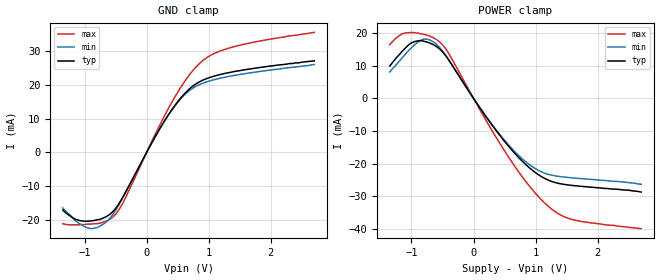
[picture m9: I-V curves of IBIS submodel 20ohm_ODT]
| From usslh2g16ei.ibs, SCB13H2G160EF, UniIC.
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| SUBMODEL 20ohm_ODT
[Submodel]   20ohm_ODT
Submodel_type  Dynamic_clamp
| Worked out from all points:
|   GND clamp passes 1 mA (typ) near -0.03 V on its own axis
[GND Clamp]
|Voltage   I(typ)   I(min)   I(max)
-1.35V    -17.1mA    -16.5mA    -21.15mA
-1.15V    -19.8mA    -20.2mA    -21.46mA
-950mV    -20.4mA    -22.4mA    -21.25mA
-650mV    -19.03mA   -20.58mA   -20.39mA
-500mV    -16.62mA   -17.18mA   -18.34mA
-400mV    -13.77mA   -13.96mA   -15.54mA
100mV     3.414mA    3.411mA    3.926mA
400mV     12.47mA    12.37mA    14.66mA
650mV     18.12mA    17.72mA    21.99mA
900mV     21.34mA    20.45mA    27.11mA
1.45V     24.05mA    22.9mA     31.49mA
2.7V      27.1mA     26mA       35.52mA
[POWER Clamp]
|Voltage   I(typ)   I(min)   I(max)
-1.35V    9.9mA      8.1mA      16.46mA
-1.15V    14.4mA     12.4mA     19.79mA
-1V       17mA       15.5mA     20.21mA
-850mV    17.7mA     17.8mA     19.79mA
-700mV    16.92mA    17.86mA    19.04mA
-550mV    15.2mA     15.66mA    17.35mA
-400mV    11.77mA    11.79mA    13.78mA
500mV     -13.18mA   -12.83mA   -16.1mA
850mV     -20.42mA   -19.55mA   -25.66mA
1.15V     -24.56mA   -22.93mA   -32.12mA
1.6V      -26.68mA   -24.35mA   -37.15mA
2.7V      -28.7mA    -26.3mA    -39.9mA
